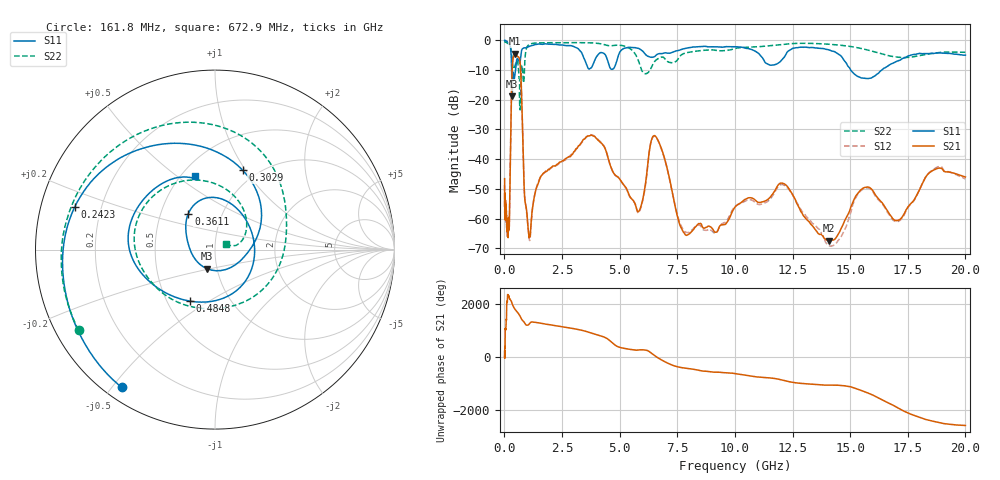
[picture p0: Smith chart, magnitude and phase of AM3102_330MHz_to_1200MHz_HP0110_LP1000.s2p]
! Date/Time: Tue, Sep 11, 2018 5:15 PM
! Network Analyzer: Agilent Technologies E8362B Rev: A.07.50.63
! Sweep from 0.010 to 20.000 GHz, 1601 Points, Sweep Type: LOG
! Power Supply: 4.949 V, 0.001 A
# Hz S DB R 50
!freq MagS11 AngS11 MagS21 AngS21 MagS12 AngS12 MagS22 AngS22
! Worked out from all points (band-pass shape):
!   1601 points, 10 MHz to 20 GHz, reference 50 ohm
!   highest |S21| = -4.43 dB at 464.5 MHz (marker M1); lowest = -67.4 dB at 14.07 GHz (marker M2)
!   |S21| within 3 dB of the highest: 354.6 MHz to 680.5 MHz (325.9 MHz wide, 63 % of centre)
!   lowest |S11| = -18.8 dB at 337.9 MHz (marker M3), VSWR 1.26, Z = 44.8 - j9.67 ohm
!   |S11| at or under -10 dB: 315 MHz to 483.8 MHz (168.8 MHz wide, 42.3 % of centre); 15.03 GHz to 16.37 GHz (1.342 GHz wide, 8.55 % of centre)
!   |S22| runs from -23.4 to -0.3 dB; largest |S21 - S12| = 0.011
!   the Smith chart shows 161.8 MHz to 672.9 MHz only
!   S11 on the Smith chart (normalised r, x): 161.8 MHz: 0.05, -0.53; 242.3 MHz: 0.10, +0.15; 302.9 MHz: 0.85, +0.97; 361.1 MHz: 0.69, +0.30; 484.8 MHz: 0.65, -0.42; 672.9 MHz: 0.59, +0.58
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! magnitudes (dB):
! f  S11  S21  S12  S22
! 10 MHz  0.0  -46.6  -48.8  -0.3
! 35.55 MHz  0.0  -58.1  -58.4  -0.5
! 126.4 MHz  -0.4  -64.4  -62.3  -0.9
! 161.8 MHz  -0.7  -65.9  -64.0  -1.1
! 242.3 MHz  -1.8  -48.6  -48.9  -1.8
! 302.9 MHz  -6.6  -20.0  -20.1  -3.6
! 337.9 MHz  -18.8  -9.5  -9.6  -6.7
! 361.1 MHz  -12.0  -6.9  -7.0  -8.3
! 447.2 MHz  -12.2  -4.4  -4.5  -8.9
! 464.5 MHz  -11.2  -4.4  -4.4  -8.4
! 484.8 MHz  -9.9  -4.5  -4.5  -7.9
! 672.9 MHz  -7.5  -6.9  -7.0  -23.2
! 869.7 MHz  -2.5  -51.7  -51.5  -10.1
! 1.072 GHz  -2.0  -66.3  -66.6  -1.4
! 1.59 GHz  -1.3  -45.7  -45.7  -0.8
! 3.793 GHz  -9.0  -32.0  -31.8  -0.8
! 5.652 GHz  -2.4  -54.7  -54.7  -4.3
! 6.58 GHz  -5.0  -32.5  -32.6  -6.6
! 7.845 GHz  -2.7  -65.4  -64.6  -4.3
! 12.09 GHz  -6.1  -48.1  -48.6  -1.3
! 14.07 GHz  -3.2  -67.4  -69.1  -1.3
! 20 GHz  -5.0  -46.0  -46.7  -4.0
